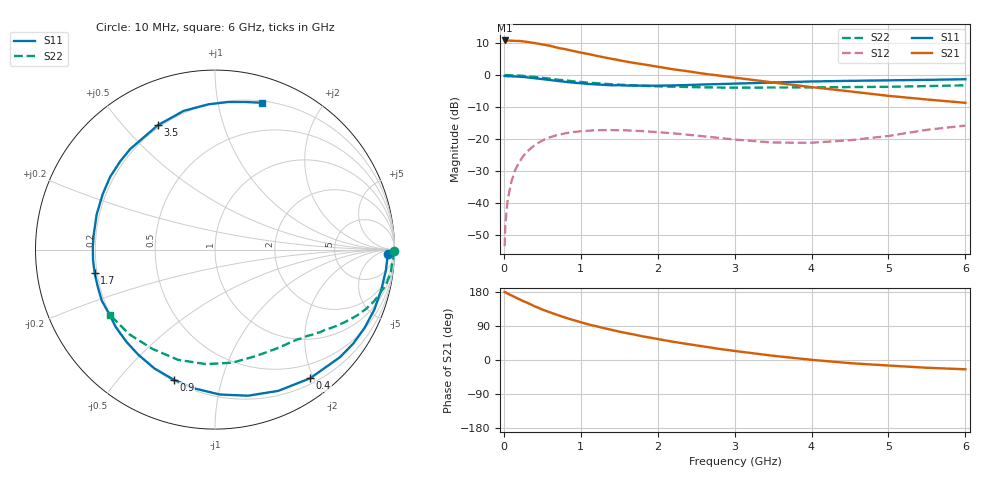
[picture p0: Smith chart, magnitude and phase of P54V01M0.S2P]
! SIEMENS Small Signal Semiconductors
! BFP183
! Si NPN RF Bipolar Junction Transistor in SOT143
! VCE = 4 V  IC = 1 mA
! Common Emitter S-Parameters:  March  1996
# GHz  S  MA  R  50
!  f  S11  S21  S12  S22
! GHz  MAG  ANG  MAG  ANG  MAG  ANG  MAG  ANG
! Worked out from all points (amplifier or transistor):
!   36 points, 10 MHz to 6 GHz, reference 50 ohm
!   highest |S21| = 10.8 dB at 10 MHz (marker M1)
!   |S21| within 3 dB of that: start of sweep to 848.3 MHz
!   unconditionally stable (mu >= 1): 2.494 GHz to end of sweep
!   at 250 MHz: K = 0.10, MSG = 18.0 dB, |S12| = -25.5 dB
!   at 1.4 GHz: K = 0.54, MSG = 11.2 dB, |S12| = -17.2 dB
!   at 6 GHz: K = 1.04, MAG = 2.3 dB, |S12| = -15.8 dB
!   S11 on the Smith chart (normalised r, x): 10 MHz: 38, -26; 400 MHz: 0.28, -1.95; 900 MHz: 0.21, -0.71; 1.7 GHz: 0.19, -0.09; 3.5 GHz: 0.19, +0.62; 6 GHz: 0.22, +1.35
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0.01  0.9645 -1.4  3.472 179.3  0.0021 90.0  0.9999 -0.5
0.02  0.9619 -2.7  3.454 178.7  0.0047 89.2  0.9972 -0.9
0.05  0.959 -6.9  3.471 175.1  0.0112 87.1  0.9953 -2.3
0.1  0.9534 -13.5  3.443 170.3  0.0219 81.8  0.9892 -4.8
0.2  0.9407 -27.6  3.416 160.4  0.0435 73.5  0.9798 -9.4
0.3  0.9188 -40.7  3.295 151.5  0.0631 65.5  0.9573 -13.8
0.4  0.8916 -53.5  3.163 141.8  0.0799 58.1  0.9333 -17.8
0.5  0.8626 -65.8  3.007 133.2  0.0945 50.9  0.9034 -21.5
0.6  0.8347 -77.2  2.87 125.7  0.1064 44.6  0.8749 -24.6
0.7  0.8079 -88.1  2.664 118.6  0.1153 39.2  0.8468 -27.4
0.8  0.7823 -98.1  2.534 111.8  0.1225 34.1  0.8224 -29.8
0.9  0.7604 -107.6  2.379 105.6  0.1283 29.3  0.7991 -32.1
1.1  0.7251 -126.1  2.13 93.9  0.1345 21.1  0.7586 -36.1
1.4  0.6901 -148.9  1.793 79.6  0.1375 11.2  0.7177 -41.5
1.7  0.6833 -168.9  1.541 66.9  0.1341 4.3  0.6867 -46.3
1.9  0.6808 178.8  1.412 59.1  0.1301 0.6  0.6716 -49.4
2.2  0.6878 163.5  1.228 48.2  0.1224 -3.7  0.6569 -54.5
2.8  0.7213 137.2  0.979 29.3  0.1037 -6.2  0.637 -66.0
3.5  0.7626 114.7  0.764 11.2  0.0879 0.8  0.6375 -81.3
4.5  0.8105 92.5  0.554 -8.3  0.0955 20.0  0.6476 -108.6
5.5  0.84 78.2  0.414 -20.5  0.139 27.1  0.6712 -135.4
6  0.8586 72.3  0.367 -24.5  0.1616 24.2  0.6896 -148.2
